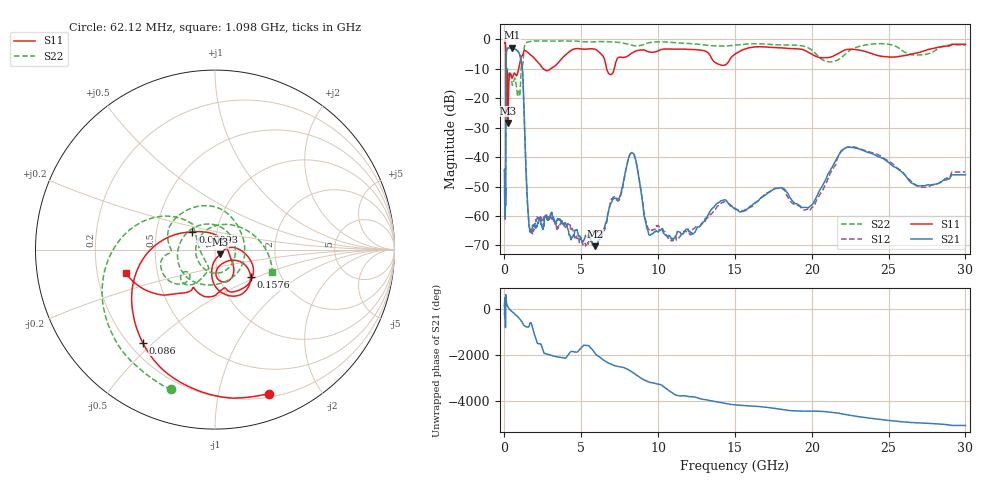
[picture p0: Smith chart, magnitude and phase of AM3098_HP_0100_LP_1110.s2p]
! Date/Time: Thu, Feb 28, 2019 8:35 AM
! Network Analyzer: Agilent Technologies E8364B Rev: A.07.50.67
! Sweep from 0.010 to 30.000 GHz, 1601 Points, Sweep Type: LOG
! Power Supply: 5.022 V, 0.002 A
# Hz S DB R 50
!freq MagS11 AngS11 MagS21 AngS21 MagS12 AngS12 MagS22 AngS22
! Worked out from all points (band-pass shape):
!   1601 points, 10 MHz to 30 GHz, reference 50 ohm
!   highest |S21| = -2.80 dB at 493.1 MHz (marker M1); lowest = -70.2 dB at 5.9 GHz (marker M2)
!   |S21| within 3 dB of the highest: 112.4 MHz to 1.028 GHz (916 MHz wide, 161 % of centre)
!   lowest |S11| = -28.4 dB at 235.1 MHz (marker M3), VSWR 1.08, Z = 52.8 - j2.74 ohm
!   |S11| at or under -10 dB: 95.96 MHz to 922.8 MHz (826.9 MHz wide, 162 % of centre); 2.534 GHz to 3.001 GHz (467.1 MHz wide, 16.9 % of centre); 6.652 GHz to 7.145 GHz (493.2 MHz wide, 7.15 % of centre)
!   |S22| runs from -22.2 to -0.5 dB; largest |S21 - S12| = 0.011
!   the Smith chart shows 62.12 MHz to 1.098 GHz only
!   S11 on the Smith chart (normalised r, x): 62.12 MHz: 0.23, -1.42; 86 MHz: 0.25, -0.46; 98.93 MHz: 0.76, +0.16; 157.6 MHz: 1.41, -0.46; 1.098 GHz: 0.33, -0.12
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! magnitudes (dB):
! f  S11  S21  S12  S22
! 10 MHz  -0.4  -48.1  -45.3  -0.6
! 38.04 MHz  -0.5  -59.6  -59.7  -1.0
! 62.12 MHz  -1.3  -50.9  -50.7  -1.8
! 76.26 MHz  -2.1  -55.6  -51.9  -2.5
! 86 MHz  -3.7  -38.2  -37.8  -4.0
! 98.93 MHz  -15.9  -12.9  -12.9  -20.1
! 144.7 MHz  -16.7  -3.6  -3.6  -13.5
! 157.6 MHz  -12.0  -3.5  -3.4  -11.3
! 235.1 MHz  -28.4  -2.9  -2.9  -12.0
! 309.6 MHz  -12.7  -2.9  -2.8  -11.3
! 493.1 MHz  -13.1  -2.8  -2.8  -15.3
! 550.5 MHz  -12.5  -3.0  -2.9  -15.1
! 1.098 GHz  -5.8  -7.6  -7.6  -9.3
! 1.59 GHz  -4.7  -62.7  -62.5  -0.8
! 2.084 GHz  -7.1  -63.8  -61.3  -0.5
! 5.9 GHz  -3.3  -70.2  -65.7  -0.8
! 7.926 GHz  -5.9  -43.6  -43.7  -1.5
! 9.443 GHz  -4.3  -66.5  -64.7  -1.1
! 10.97 GHz  -3.3  -67.9  -68.4  -1.1
! 19.7 GHz  -4.2  -57.2  -57.7  -2.7
! 22.67 GHz  -3.4  -36.7  -36.5  -3.2
! 30 GHz  -1.7  -46.0  -45.0  -1.9
